TYPE dut_EXH_Input :
STRUCT

	I300_00			:BOOL;	//	FS105_RHC_Flow_Alarm
	I300_01			:BOOL;	//	FS106_Heater_Jacket_Flow_Alarm
	I300_02			:BOOL;	//	FS202_Heater_Upper_Alarm
	I300_03			:BOOL;	//	FS104_Shutter_Flow_Alarm
	I300_04			:BOOL;	//	FS111_BoatRotation_Flow_Alarm
	I300_05			:BOOL;	//	FS102_Flange_Flow_Alarm
	I300_06			:BOOL;	//	Spare
	I300_07			:BOOL;	//	Spare
	I300_08			:BOOL;	//	VG11_Status_OK
	I300_09			:BOOL;	//	VG11_Low_Alarm
	I300_10			:BOOL;	//	VG11_High_Alarm
	I300_11			:BOOL;	//	VG13_Status_OK
	I300_12			:BOOL;	//	VG13_Low_Alarm
	I300_13			:BOOL;	//	VG13_High_Alarm
	I300_14			:BOOL;	//	AV71_Fan1_Alarm
	I300_15			:BOOL;	//	AV71_Fan2_Alarm
	I301_00			:BOOL;	//	DG1_Low_Limit_Alarm
	I301_01			:BOOL;	//	DG1_High_Limit_Alarm
	I301_02			:BOOL;	//	Spare
	I301_03			:BOOL;	//	Spare
	I301_04			:BOOL;	//	Spare
	I301_05			:BOOL;	//	Spare
	I301_06			:BOOL;	//	Spare
	I301_07			:BOOL;	//	Spare
	I301_08			:BOOL;	//	MP/PS21_Pressure_Low_Alarm
	I301_09			:BOOL;	//	FS101_MainWater_Flow_Alarm-1
	I301_10			:BOOL;	//	FS101_FMainWater_low_Alarm-2
	I301_11			:BOOL;	//	FL301_Flow_Switch
	I301_12			:BOOL;	//	Spare
	I301_13			:BOOL;	//	FS116_Zaxis_Flow_Alarm
	I301_14			:BOOL;	//	PS110_Pressure_Low_Alarm
	I301_15			:BOOL;	//	PS110_Pressure_High_Alarm
	I302_00			:BOOL;	//	PG/PS12_Pressure_Low_Alarm
	I302_01			:BOOL;	//	PG/PS12_Pressure_High_Alarm
	I302_02			:BOOL;	//	PS13_ATM_Status
	I302_03			:BOOL;	//	PS13_High_Limit_Alarm
	I302_04			:BOOL;	//	PG101_Water_Pressure_Low_Alarm
	I302_05			:BOOL;	//	PG101_Water_Pressure_High_Alarm
	I302_06			:BOOL;	//	VG14_Status_OK
	I302_07			:BOOL;	//	VG14_LOW_Alarm
	I302_08			:BOOL;	//	VG14_High_Alarm
	I302_09			:BOOL;	//	PS14_Pressure_Low_Alarm
	I302_10			:BOOL;	//	PS14_Pressure_High_Alarm
	I302_11			:BOOL;	//	Spare
	I302_12			:BOOL;	//	Spare
	I302_13			:BOOL;	//	Spare
	I302_14			:BOOL;	//	Spare
	I302_15			:BOOL;	//	Spare
	I303_00			:BOOL;	//	APC_Valve_Status
	I303_01			:BOOL;	//	APC_Alarm_Status
	I303_02			:BOOL;	//	RHC_Cooling_Air_cylinder1_Open
	I303_03			:BOOL;	//	RHC_Cooling_Air_cylinder1_Close
	I303_04			:BOOL;	//	RHC_Cooling_Air_cylinder2_Open
	I303_05			:BOOL;	//	RHC_Cooling_Air_cylinder2_Close
	I303_06			:BOOL;	//	RHC_Cooling_Valve_Open
	I303_07			:BOOL;	//	RHC_Cooling_Valve_Close
	I303_08			:BOOL;	//	RHC_Cooling_ButterflyValves_Open
	I303_09			:BOOL;	//	RHC_Cooling_ButterflyValves_Close
	I303_10			:BOOL;	//	Spare
	I303_11			:BOOL;	//	Spare
	I303_12			:BOOL;	//	GV_Open_NC
	I303_13			:BOOL;	//	GV_Open_NO
	I303_14			:BOOL;	//	GV_Close_NC
	I303_15			:BOOL;	//	GV_Close_NO
	I304_00			:BOOL;	//	RHC_Cooling_BallValve_Open
	I304_01			:BOOL;	//	RHC_Cooling_BallValve_Close
	I304_02			:BOOL;	//	Spare
	I304_03			:BOOL;	//	Spare
	I304_04			:BOOL;	//	Spare
	I304_05			:BOOL;	//	Spare
	I304_06			:BOOL;	//	Spare
	I304_07			:BOOL;	//	Spare
	I304_08			:BOOL;	//	Spare
	I304_09			:BOOL;	//	Spare
	I304_10			:BOOL;	//	Spare
	I304_11			:BOOL;	//	Spare
	I304_12			:BOOL;	//	Spare
	I304_13			:BOOL;	//	Spare
	I304_14			:BOOL;	//	Spare
	I304_15			:BOOL;	//	Spare	

	IW300			:INT;	//	FS105_RHC_Colling_Water_Flow
	IW301			:INT;	//	FS106_Heater_Jacket_Cooling_Water_Flow
	IW302			:INT;	//	FS202_Furnace_Cooling_Water_Flow
	IW303			:INT;	//	FS104_Shutter_Cooling_Water_Flow
	IW304			:INT;	//	FS111_Boat_Rotation_Cooling_Water_Flow
	IW305			:INT;	//	FS102_Flange_Cooling_Water_Flow
	IW306			:INT;	//	SPARE
	IW307			:INT;	//	SPARE
	IW308			:INT;	//	DG1_Pressure
	IW309			:INT;	//	SPARE
	IW310			:INT;	//	SPARE
	IW311			:INT;	//	FS116_Radiator_Cooling_Water_Flow
	IW312			:INT;	//	PS13_Pressure
	IW313			:INT;	//	SPARE
	IW314			:INT;	//	SPARE
	IW315			:INT;	//	SPARE
	IW316			:INT;	//	SPARE
	IW317			:INT;	//	SPARE
	IW318			:INT;	//	PS21_Pressure
	IW319			:INT;	//	PS110_Pressure
	IW320			:INT;	//	PG/PS12_Pressure
	IW321			:INT;	//	VG14_Pressure
	IW322			:INT;	//	PS14_Pressure
	IW323			:INT;	//	SPARE
	IW324			:INT;	//	SPARE
	IW325			:INT;	//	SPARE
	IW326			:INT;	//	SPARE
	IW327			:INT;	//	SPARE
	IW328			:INT;	//	SPARE
	IW329			:INT;	//	SPARE
	IW330			:INT;	//	SPARE
	IW331			:INT;	//	SPARE
	IW332			:INT;	//	spare
	IW333			:INT;	//	SPARE
	IW334			:INT;	//	SPARE
	IW335			:INT;	//	SPARE

END_STRUCT
END_TYPE
